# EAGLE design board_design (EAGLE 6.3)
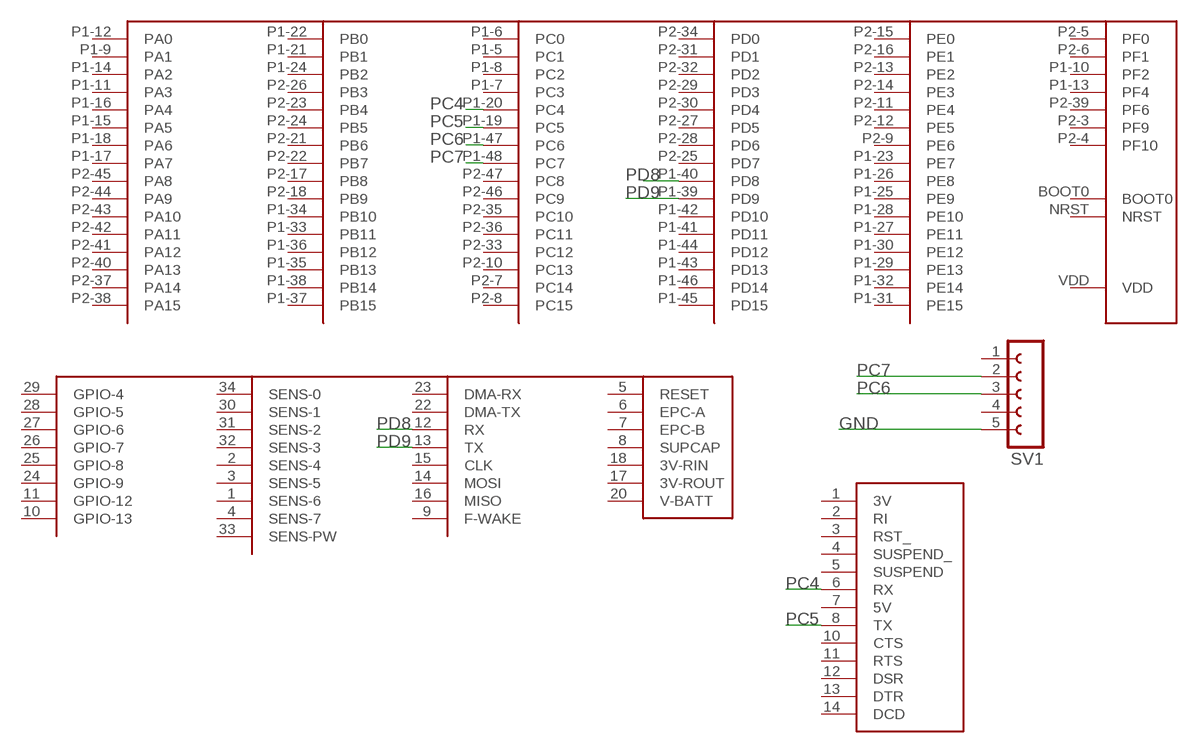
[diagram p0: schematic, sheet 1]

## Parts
M2  USB_SER  [USB_SER]
ST1  STM32_F3  [STM32F3]
SV1  FE05-1  [FE05-1]
U$1  WIFLY-RN-131C  [DIL34-11]

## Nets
GND: SV1.5
PC4: M2.6(RX) ST1.P1-20(PC4)
PC5: M2.8(TX) ST1.P1-19(PC5)
PC6: ST1.P1-47(PC6) SV1.3
PC7: ST1.P1-48(PC7) SV1.2
PD8: ST1.P1-40(PD8) U$1.12(RX)
PD9: ST1.P1-39(PD9) U$1.13(TX)
Unconnected: M2.1(3V) M2.2(RI) M2.3(RST_) M2.4(SUSPEND_) M2.5(SUSPEND) M2.7(5V) M2.10(CTS) M2.11(RTS) M2.12(DSR) M2.13(DTR) M2.14(DCD) ST1.BOOT0 ST1.NRST ST1.P1-5(PC1) ST1.P1-6(PC0) ST1.P1-7(PC3) ST1.P1-8(PC2) ST1.P1-9(PA1) ST1.P1-10(PF2) ST1.P1-11(PA3) ST1.P1-12(PA0) ST1.P1-13(PF4) ST1.P1-14(PA2) ST1.P1-15(PA5) ST1.P1-16(PA4) ST1.P1-17(PA7) ST1.P1-18(PA6) ST1.P1-21(PB1) ST1.P1-22(PB0) ST1.P1-23(PE7) ST1.P1-24(PB2) ST1.P1-25(PE9) ST1.P1-26(PE8) ST1.P1-27(PE11) ST1.P1-28(PE10) ST1.P1-29(PE13) ST1.P1-30(PE12) ST1.P1-31(PE15) ST1.P1-32(PE14) ST1.P1-33(PB11) ST1.P1-34(PB10) ST1.P1-35(PB13) ST1.P1-36(PB12) ST1.P1-37(PB15) ST1.P1-38(PB14) ST1.P1-41(PD11) ST1.P1-42(PD10) ST1.P1-43(PD13) ST1.P1-44(PD12) ST1.P1-45(PD15) ST1.P1-46(PD14) ST1.P2-3(PF9) ST1.P2-4(PF10) ST1.P2-5(PF0) ST1.P2-6(PF1) ST1.P2-7(PC14) ST1.P2-8(PC15) ST1.P2-9(PE6) ST1.P2-10(PC13) ST1.P2-11(PE4) ST1.P2-12(PE5) ST1.P2-13(PE2) ST1.P2-14(PE3) ST1.P2-15(PE0) ST1.P2-16(PE1) ST1.P2-17(PB8) ST1.P2-18(PB9) ST1.P2-21(PB6) ST1.P2-22(PB7) ST1.P2-23(PB4) ST1.P2-24(PB5) ST1.P2-25(PD7) ST1.P2-26(PB3) ST1.P2-27(PD5) ST1.P2-28(PD6) ST1.P2-29(PD3) ST1.P2-30(PD4) ST1.P2-31(PD1) ST1.P2-32(PD2) ST1.P2-33(PC12) ST1.P2-34(PD0) ST1.P2-35(PC10) ST1.P2-36(PC11) ST1.P2-37(PA14) ST1.P2-38(PA15) ST1.P2-39(PF6) ST1.P2-40(PA13) ST1.P2-41(PA12) ST1.P2-42(PA11) ST1.P2-43(PA10) ST1.P2-44(PA9) ST1.P2-45(PA8) ST1.P2-46(PC9) ST1.P2-47(PC8) SV1.1 SV1.4 U$1.1(SENS-6) U$1.2(SENS-4) U$1.3(SENS-5) U$1.4(SENS-7) U$1.5(RESET) U$1.6(EPC-A) U$1.7(EPC-B) U$1.8(SUPCAP) U$1.9(F-WAKE) U$1.10(GPIO-13) U$1.11(GPIO-12) U$1.14(MOSI) U$1.15(CLK) U$1.16(MISO) U$1.17(3V-ROUT) U$1.18(3V-RIN) U$1.20(V-BATT) U$1.22(DMA-TX) U$1.23(DMA-RX) U$1.24(GPIO-9) U$1.25(GPIO-8) U$1.26(GPIO-7) U$1.27(GPIO-6) U$1.28(GPIO-5) U$1.29(GPIO-4) U$1.30(SENS-1) U$1.31(SENS-2) U$1.32(SENS-3) U$1.33(SENS-PW) U$1.34(SENS-0)

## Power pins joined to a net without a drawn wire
5V: ST1.5V-A(5V) ST1.5V-B(5V)
GND: M2.9(GND) ST1.GND1(GND) ST1.GND2(GND) ST1.GND3(GND) ST1.GND4(GND) ST1.GND5(GND) ST1.GND6(GND) ST1.GND7(GND) ST1.GND8(GND) ST1.GND9(GND) U$1.19(GND)
VCC: ST1.3V-A(VCC) ST1.3V-B(VCC) U$1.21(VCC)
VDD: ST1.VDD

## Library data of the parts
M2 = P442:USB_SER: USB to Serial Converter (Pololu)
ST1 = P442:STM32_F3: STM32 F3 Discovery Board
SV1 = con-lsta:FE05-1: FEMALE HEADER; OC_FARNELL: unknown; OC_NEWARK: unknown
U$1 = P442:WIFLY-RN-131C

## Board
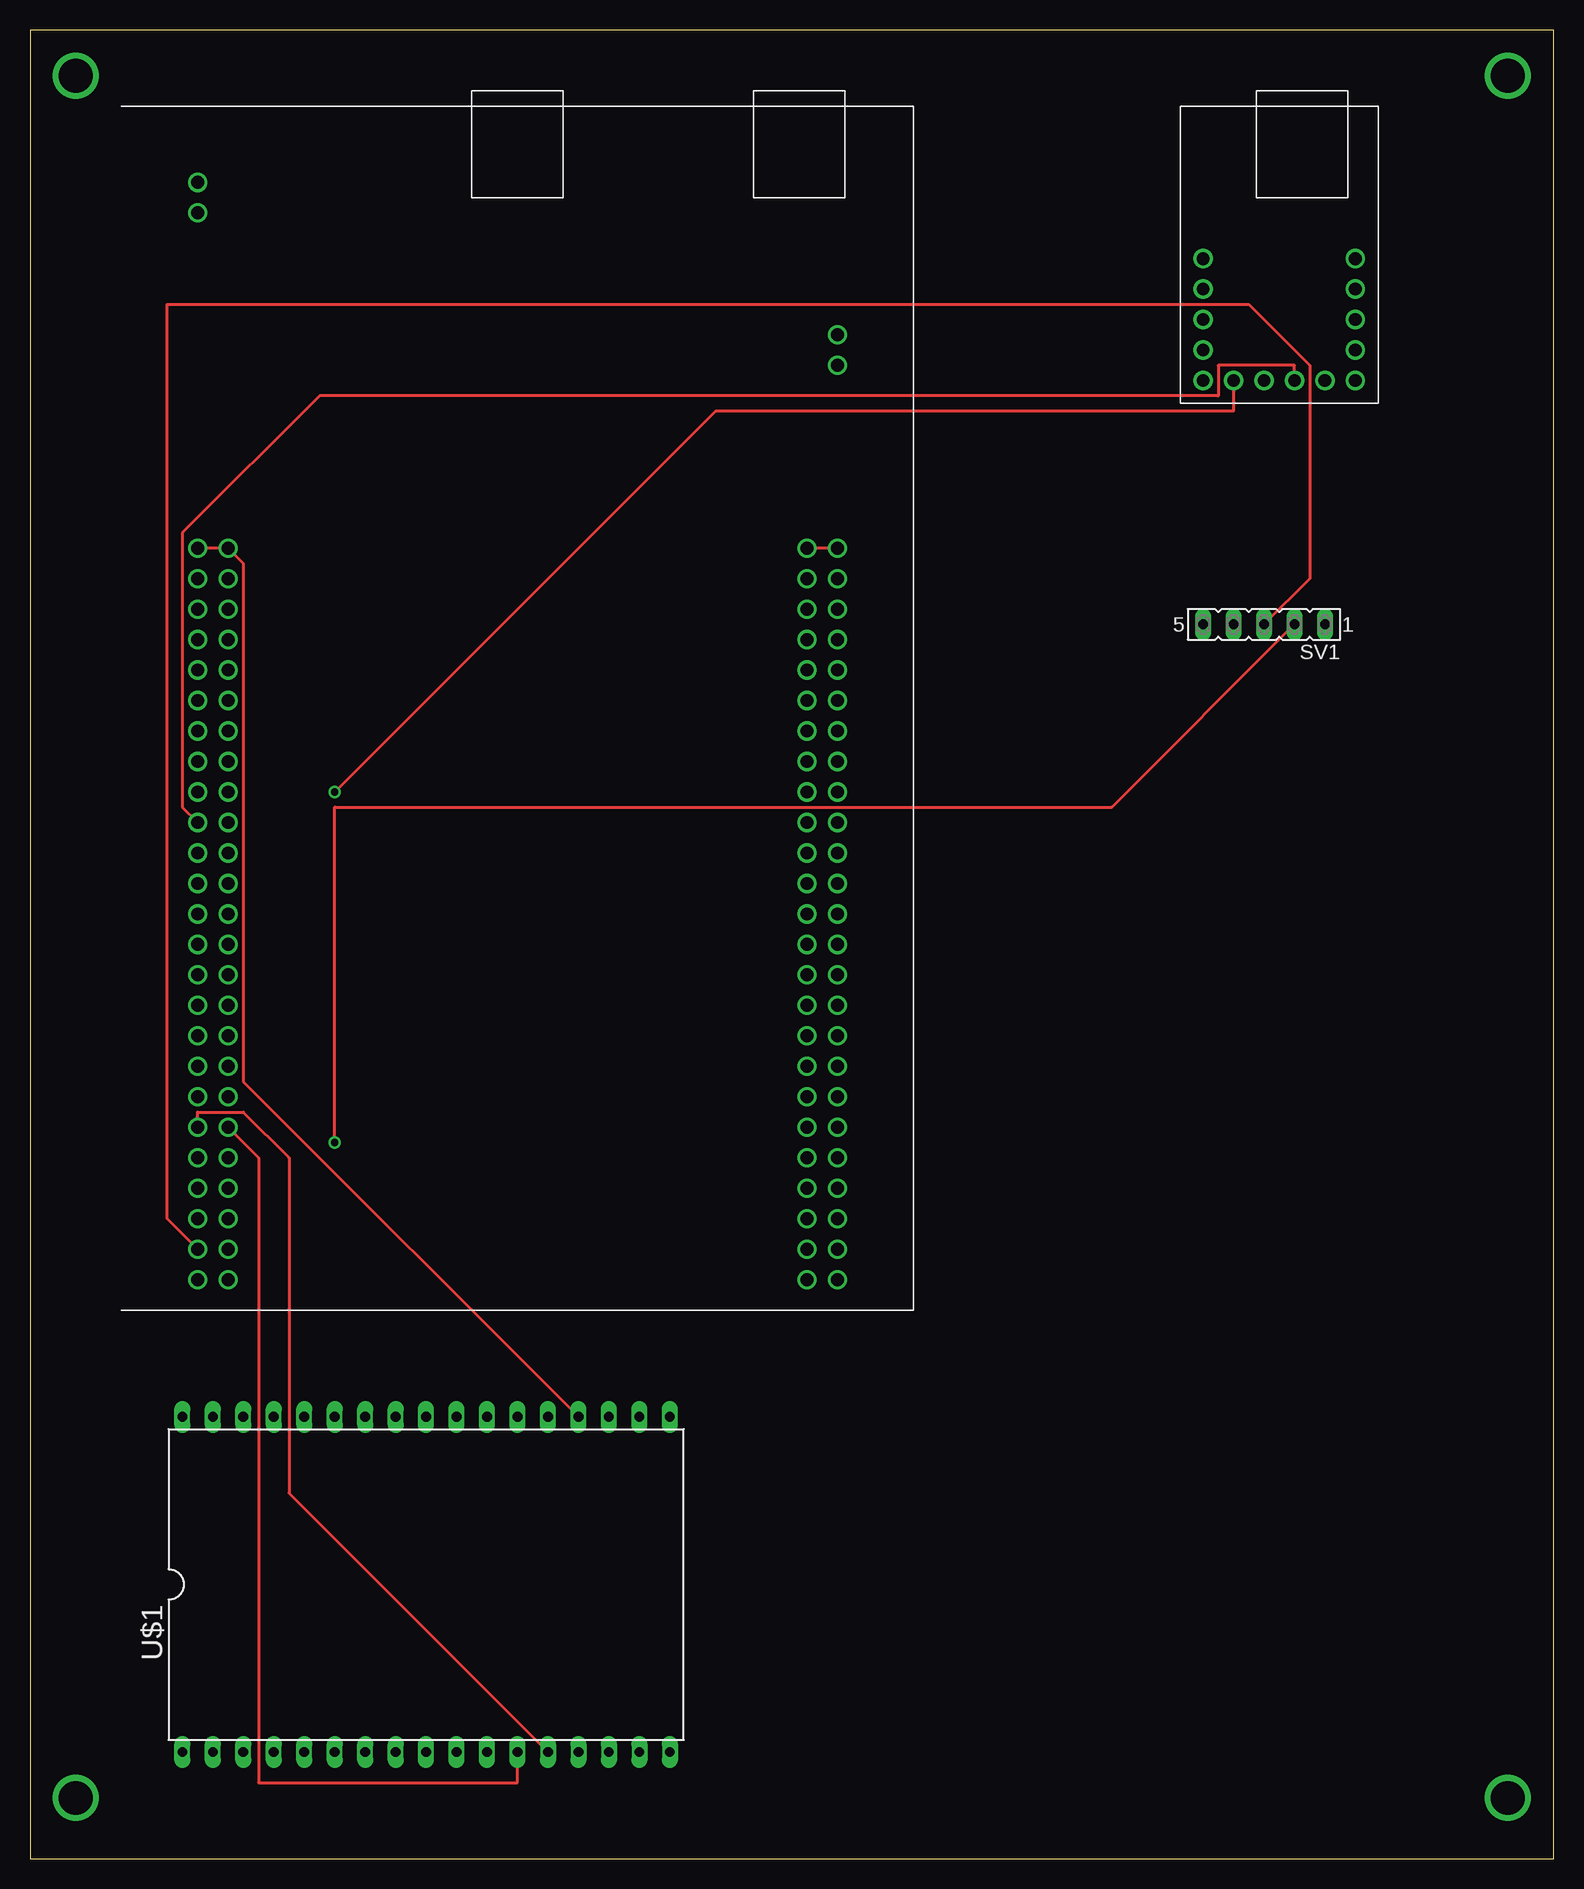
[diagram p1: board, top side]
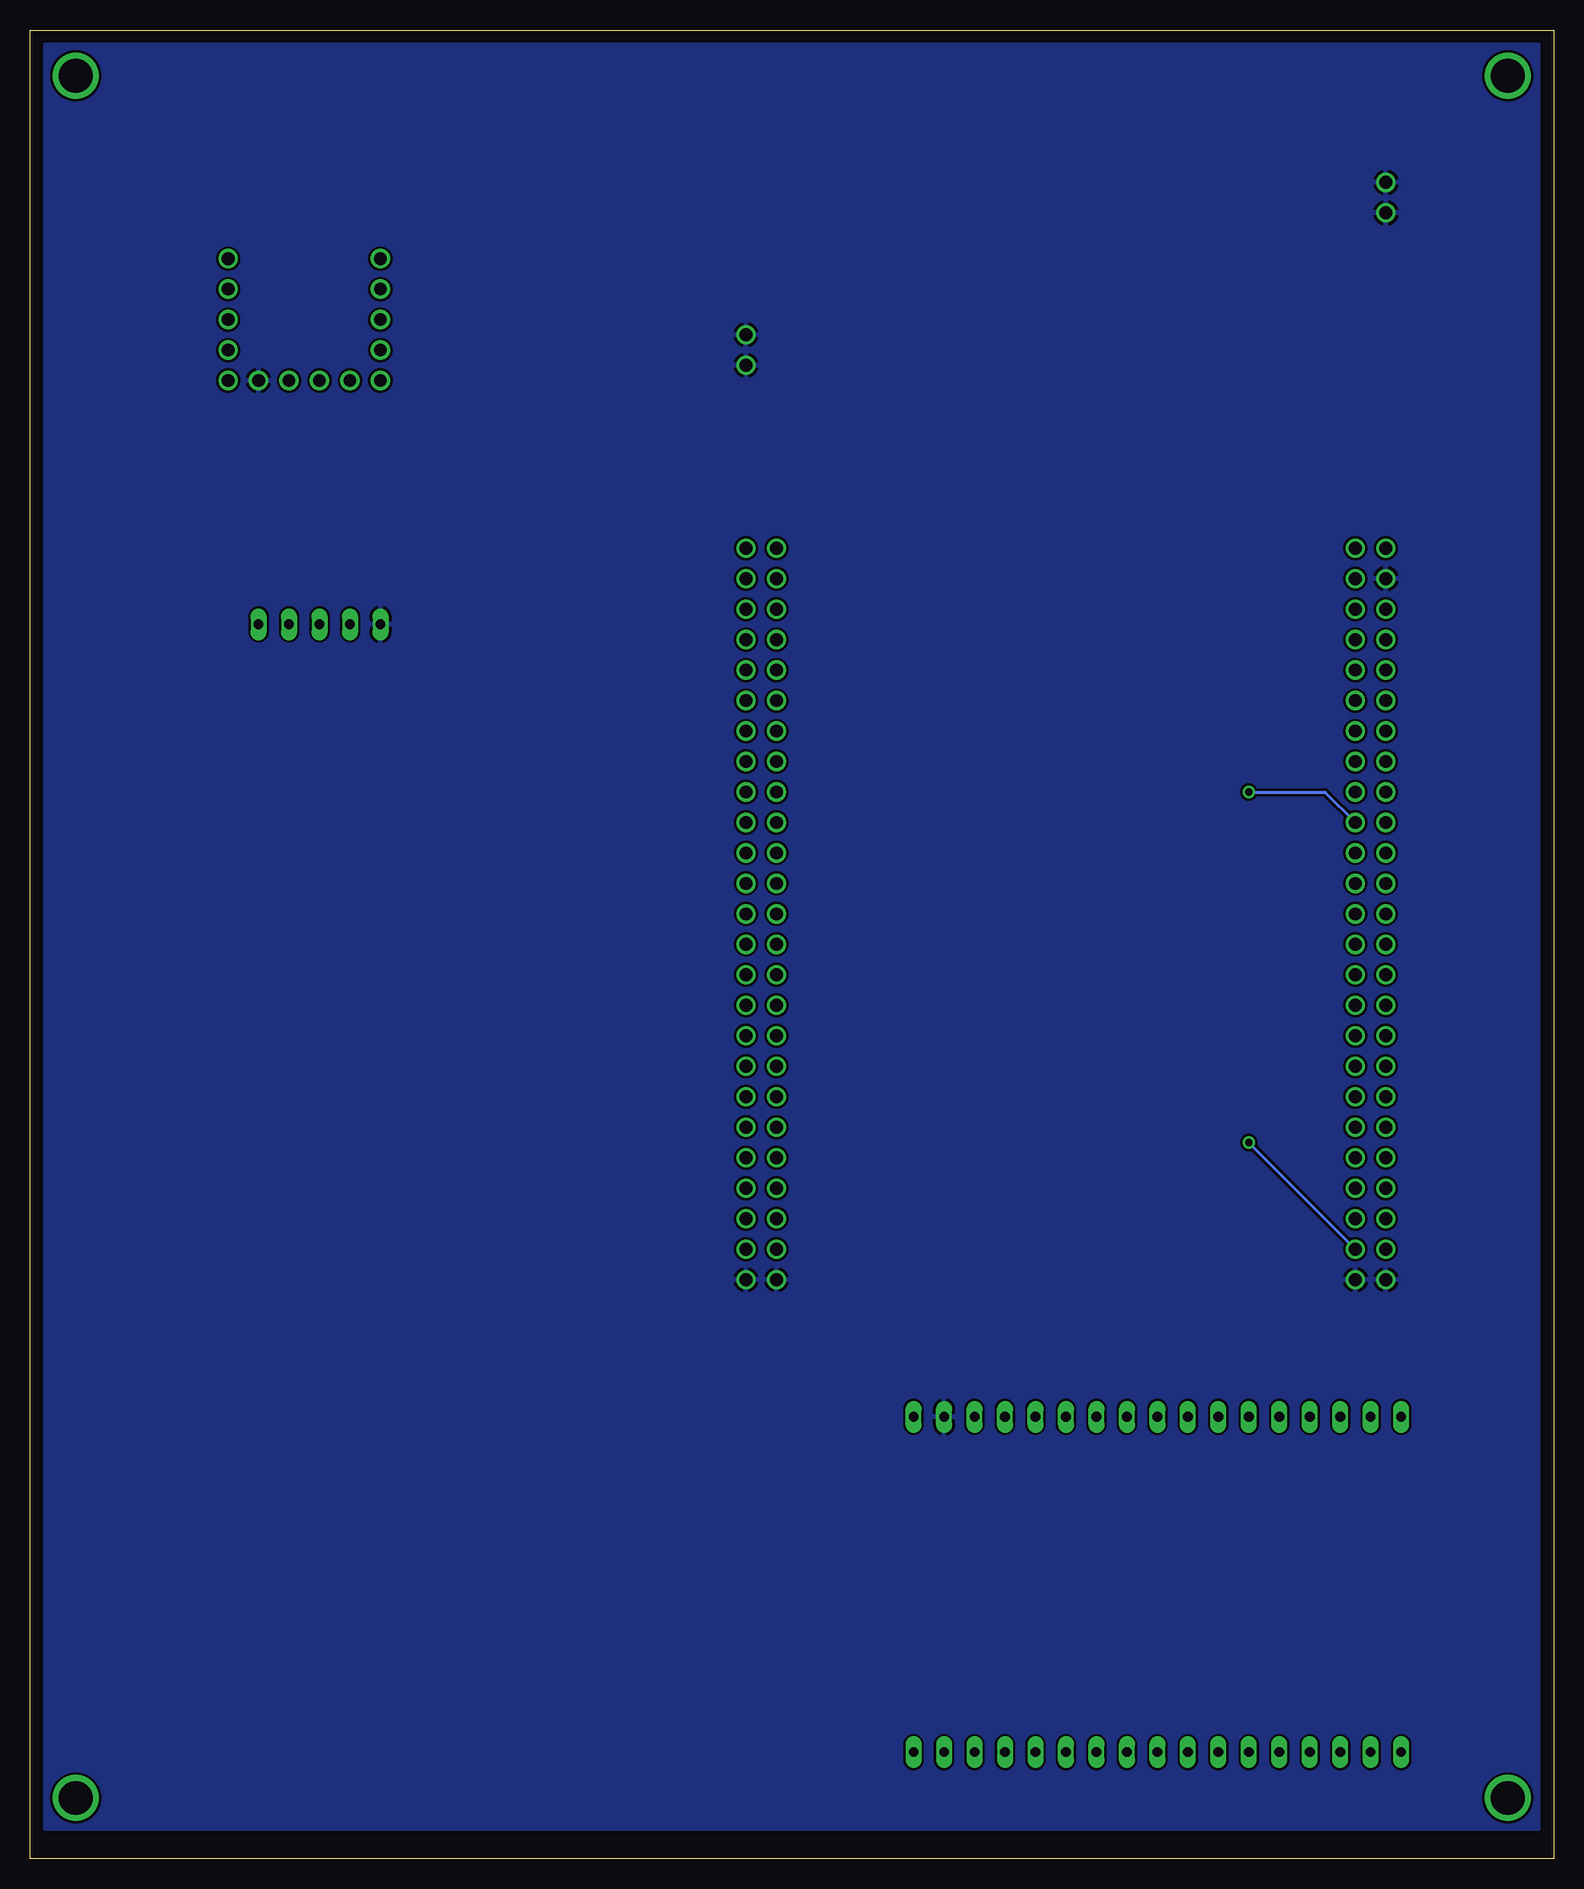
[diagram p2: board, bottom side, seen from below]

Size 127 x 152.4 mm. Coordinates in mm from the lower left corner, seen from the top.
Outline: 0,0 127,0 127,152.4 0,152.4 0,0
Copper layers (1*16): Top 0.035mm / dielectric 1.5mm / Bottom 0.035mm
Design rules "default": minimum track width 10mil, minimum drill 24mil, track to track 8mil, track to pad 8mil, pad to pad 8mil, via to via 8mil, smd to smd 8mil, copper to edge 40mil, drill to drill 8mil, minimum pad ring 10mil, minimum via ring 8mil, stop-mask expansion 4mil, vias tented up to drill 0mil, thermal gap 10mil

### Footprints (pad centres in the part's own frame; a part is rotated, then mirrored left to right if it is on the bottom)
USB_SER = drill 1.067: 1 -6.35,10.16; 2 -6.35,7.62; 3 -6.35,5.08; 4 -6.35,2.54; 5 -6.35,0; 6 -3.81,0; 7 -1.27,0; 8 1.27,0; 9 3.81,0; 10 6.35,0; 11 6.35,2.54; 12 6.35,5.08; 13 6.35,7.62; 14 6.35,10.16
STM32F3 = drill 1.067: 3V-A -26.67,60.96; 3V-B -24.13,60.96; 5V-A 24.13,60.96; 5V-B 26.67,60.96; BOOT0 24.13,38.1; GND1 -26.67,0; GND2 -24.13,0; GND3 24.13,0; GND4 26.67,0; GND5 -26.67,91.44; GND6 -26.67,88.9; GND7 26.67,78.74; GND8 26.67,76.2; GND9 -26.67,58.42; NRST -24.13,58.42; P1-5 -26.67,55.88; P1-6 -24.13,55.88; P1-7 -26.67,53.34; P1-8 -24.13,53.34; P1-9 -26.67,50.8; P1-10 -24.13,50.8; P1-11 -26.67,48.26; P1-12 -24.13,48.26; P1-13 -26.67,45.72; P1-14 -24.13,45.72; P1-15 -26.67,43.18; P1-16 -24.13,43.18; P1-17 -26.67,40.64; P1-18 -24.13,40.64; P1-19 -26.67,38.1; P1-20 -24.13,38.1; P1-21 -26.67,35.56; P1-22 -24.13,35.56; P1-23 -26.67,33.02; P1-24 -24.13,33.02; P1-25 -26.67,30.48; P1-26 -24.13,30.48; P1-27 -26.67,27.94; P1-28 -24.13,27.94; P1-29 -26.67,25.4; P1-30 -24.13,25.4; P1-31 -26.67,22.86; P1-32 -24.13,22.86; P1-33 -26.67,20.32; P1-34 -24.13,20.32; P1-35 -26.67,17.78; P1-36 -24.13,17.78; P1-37 -26.67,15.24; P1-38 -24.13,15.24; P1-39 -26.67,12.7; P1-40 -24.13,12.7; P1-41 -26.67,10.16; P1-42 -24.13,10.16; P1-43 -26.67,7.62; P1-44 -24.13,7.62; P1-45 -26.67,5.08; P1-46 -24.13,5.08; P1-47 -26.67,2.54; P1-48 -24.13,2.54; P2-3 24.13,58.42; P2-4 26.67,58.42; P2-5 24.13,55.88; P2-6 26.67,55.88; P2-7 24.13,53.34; P2-8 26.67,53.34; P2-9 24.13,50.8; P2-10 26.67,50.8; P2-11 24.13,48.26; P2-12 26.67,48.26; P2-13 24.13,45.72; P2-14 26.67,45.72; P2-15 24.13,43.18; P2-16 26.67,43.18; P2-17 24.13,40.64; P2-18 26.67,40.64; P2-21 24.13,35.56; P2-22 26.67,35.56; P2-23 24.13,33.02; P2-24 26.67,33.02; P2-25 24.13,30.48; P2-26 26.67,30.48; P2-27 24.13,27.94; P2-28 26.67,27.94; P2-29 24.13,25.4; P2-30 26.67,25.4; P2-31 24.13,22.86; P2-32 26.67,22.86; P2-33 24.13,20.32; P2-34 26.67,20.32; P2-35 24.13,17.78; P2-36 26.67,17.78; P2-37 24.13,15.24; P2-38 26.67,15.24; P2-39 24.13,12.7; P2-40 26.67,12.7; P2-41 24.13,10.16; P2-42 26.67,10.16; P2-43 24.13,7.62; P2-44 26.67,7.62; P2-45 24.13,5.08; P2-46 26.67,5.08; P2-47 24.13,2.54; P2-48 26.67,2.54; VDD 26.67,38.1
FE05-1 = drill 0.813 long: 1 -5.08,0; 2 -2.54,0; 3 0,0; 4 2.54,0; 5 5.08,0
DIL34-11 = drill 0.813 long: 1 -12.7,-13.97; 2 -10.16,-13.97; 3 -7.62,-13.97; 4 -5.08,-13.97; 5 -2.54,-13.97; 6 0,-13.97; 7 2.54,-13.97; 8 5.08,-13.97; 9 7.62,-13.97; 10 10.16,-13.97; 11 12.7,-13.97; 12 15.24,-13.97; 13 17.78,-13.97; 14 20.32,-13.97; 15 22.86,-13.97; 16 25.4,-13.97; 17 27.94,-13.97; 18 27.94,13.97; 19 25.4,13.97; 20 22.86,13.97; 21 20.32,13.97; 22 17.78,13.97; 23 15.24,13.97; 24 12.7,13.97; 25 10.16,13.97; 26 7.62,13.97; 27 5.08,13.97; 28 2.54,13.97; 29 0,13.97; 30 -2.54,13.97; 31 -5.08,13.97; 32 -7.62,13.97; 33 -10.16,13.97; 34 -12.7,13.97

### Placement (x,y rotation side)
M2  104.14,123.19 0 top
ST1  40.64,48.26 0 top
SV1  102.87,102.87 180 top
U$1  25.4,22.86 0 top

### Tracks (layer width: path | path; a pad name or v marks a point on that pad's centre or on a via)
5V
  Top 0.254: ST1.5V-B ST1.5V-A
GND
  pour Bottom: 1.27,151.13 125.73,151.13 125.73,2.54 1.27,2.54
N$5  (via drill 2.8)
  other vias: 3.81,148.59
N$6  (via drill 2.8)
  other vias: 3.81,5.08
N$7  (via drill 2.8)
  other vias: 123.19,5.08
N$8  (via drill 2.8)
  other vias: 123.19,148.59
PC4  (via drill 0.61)
  Top 0.254: v25.4,88.9 57.15,120.65 100.33,120.65 M2.6
  Bottom 0.254: ST1.P1-20 19.05,88.9 v25.4,88.9
PC5
  Top 0.254: ST1.P1-19 12.7,87.63 12.7,110.49 24.13,121.92 99.06,121.92 99.06,124.46 105.41,124.46 M2.8
PC6
  Top 0.254: SV1.3 106.68,106.68 106.68,124.46 101.6,129.54 11.43,129.54 11.43,53.34 ST1.P1-47
PC7  (via drill 0.61)
  Top 0.254: SV1.2 90.17,87.63 25.4,87.63 v25.4,59.69
  Bottom 0.254: ST1.P1-48 v25.4,59.69
PD8
  Top 0.254: ST1.P1-40 19.05,58.42 19.05,6.35 40.64,6.35 U$1.12
PD9
  Top 0.254: ST1.P1-39 13.97,62.23 17.78,62.23 21.59,58.42 21.59,30.48 U$1.13
VCC
  Top 0.254: U$1.21 17.78,64.77 17.78,107.95 ST1.3V-B ST1.3V-A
